(* Logix 5000 Routine export ReadAllSegStatus; software revision 20.04 *)

TYPE Segment_Status :
STRUCT
   Speed_pulse_status : BOOL; {access Read Only}
   Exists : BOOL; {access Read Only}
   Group_number : INT; {access Read Only}
END_STRUCT
END_TYPE

VAR_GLOBAL   (* controller tags *)
   Status_of_Segments : Segment_Status[50]; {access Read Only}
END_VAR

PROGRAM MainProgram

ROUTINE ReadAllSegStatus   (* ladder *)
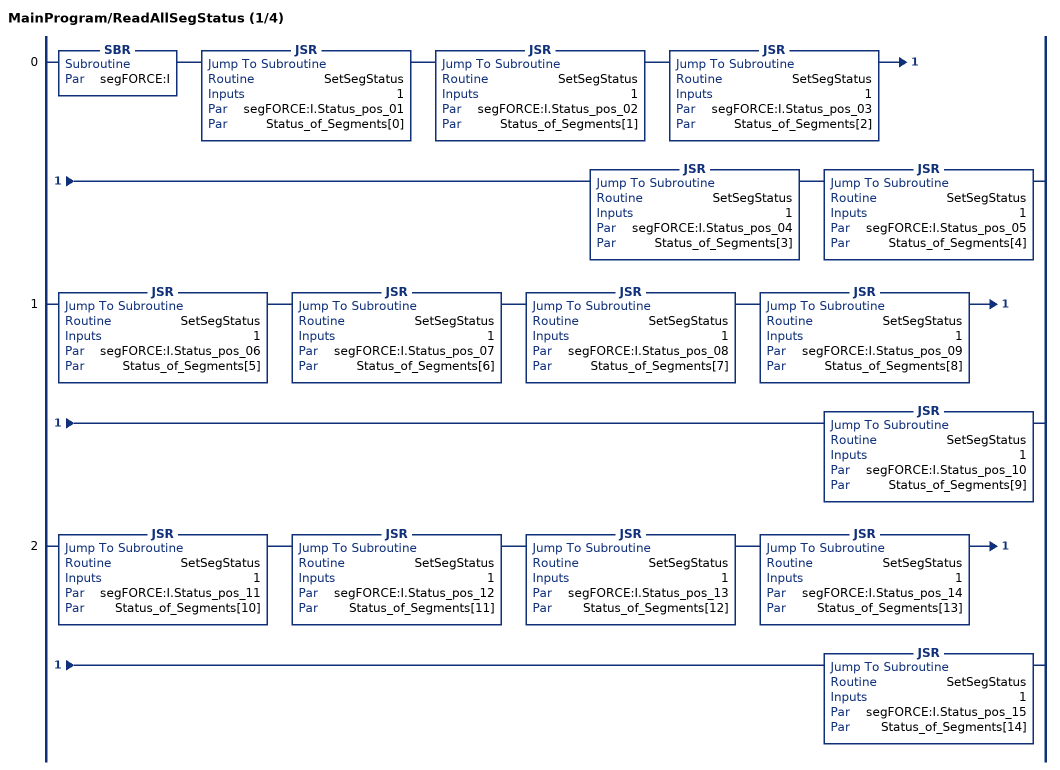
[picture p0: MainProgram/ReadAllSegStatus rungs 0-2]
   0: SBR(segFORCE:I)JSR(SetSegStatus,1,segFORCE:I.Status_pos_01,Status_of_Segments[0])JSR(SetSegStatus,1,segFORCE:I.Status_pos_02,Status_of_Segments[1])JSR(SetSegStatus,1,segFORCE:I.Status_pos_03,Status_of_Segments[2])JSR(SetSegStatus,1,segFORCE:I.Status_pos_04,Status_of_Segments[3])JSR(SetSegStatus,1,segFORCE:I.Status_pos_05,Status_of_Segments[4]);
   1: JSR(SetSegStatus,1,segFORCE:I.Status_pos_06,Status_of_Segments[5])JSR(SetSegStatus,1,segFORCE:I.Status_pos_07,Status_of_Segments[6])JSR(SetSegStatus,1,segFORCE:I.Status_pos_08,Status_of_Segments[7])JSR(SetSegStatus,1,segFORCE:I.Status_pos_09,Status_of_Segments[8])JSR(SetSegStatus,1,segFORCE:I.Status_pos_10,Status_of_Segments[9]);
   2: JSR(SetSegStatus,1,segFORCE:I.Status_pos_11,Status_of_Segments[10])JSR(SetSegStatus,1,segFORCE:I.Status_pos_12,Status_of_Segments[11])JSR(SetSegStatus,1,segFORCE:I.Status_pos_13,Status_of_Segments[12])JSR(SetSegStatus,1,segFORCE:I.Status_pos_14,Status_of_Segments[13])JSR(SetSegStatus,1,segFORCE:I.Status_pos_15,Status_of_Segments[14]);
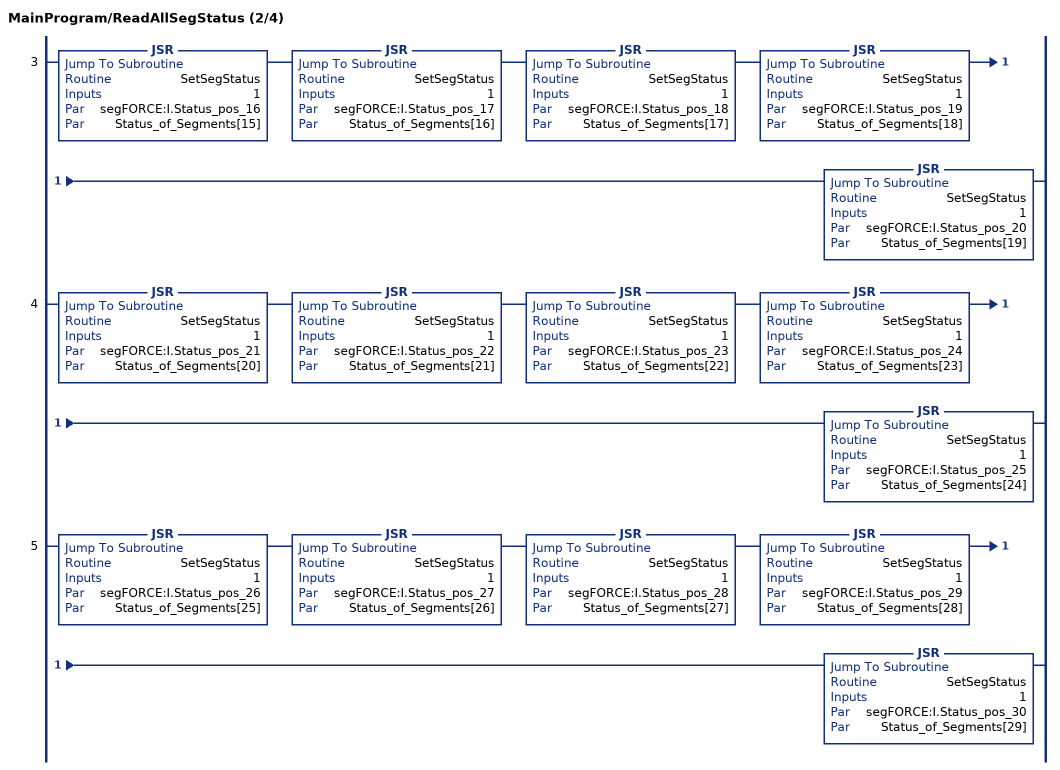
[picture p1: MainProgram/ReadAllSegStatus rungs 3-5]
   3: JSR(SetSegStatus,1,segFORCE:I.Status_pos_16,Status_of_Segments[15])JSR(SetSegStatus,1,segFORCE:I.Status_pos_17,Status_of_Segments[16])JSR(SetSegStatus,1,segFORCE:I.Status_pos_18,Status_of_Segments[17])JSR(SetSegStatus,1,segFORCE:I.Status_pos_19,Status_of_Segments[18])JSR(SetSegStatus,1,segFORCE:I.Status_pos_20,Status_of_Segments[19]);
   4: JSR(SetSegStatus,1,segFORCE:I.Status_pos_21,Status_of_Segments[20])JSR(SetSegStatus,1,segFORCE:I.Status_pos_22,Status_of_Segments[21])JSR(SetSegStatus,1,segFORCE:I.Status_pos_23,Status_of_Segments[22])JSR(SetSegStatus,1,segFORCE:I.Status_pos_24,Status_of_Segments[23])JSR(SetSegStatus,1,segFORCE:I.Status_pos_25,Status_of_Segments[24]);
   5: JSR(SetSegStatus,1,segFORCE:I.Status_pos_26,Status_of_Segments[25])JSR(SetSegStatus,1,segFORCE:I.Status_pos_27,Status_of_Segments[26])JSR(SetSegStatus,1,segFORCE:I.Status_pos_28,Status_of_Segments[27])JSR(SetSegStatus,1,segFORCE:I.Status_pos_29,Status_of_Segments[28])JSR(SetSegStatus,1,segFORCE:I.Status_pos_30,Status_of_Segments[29]);
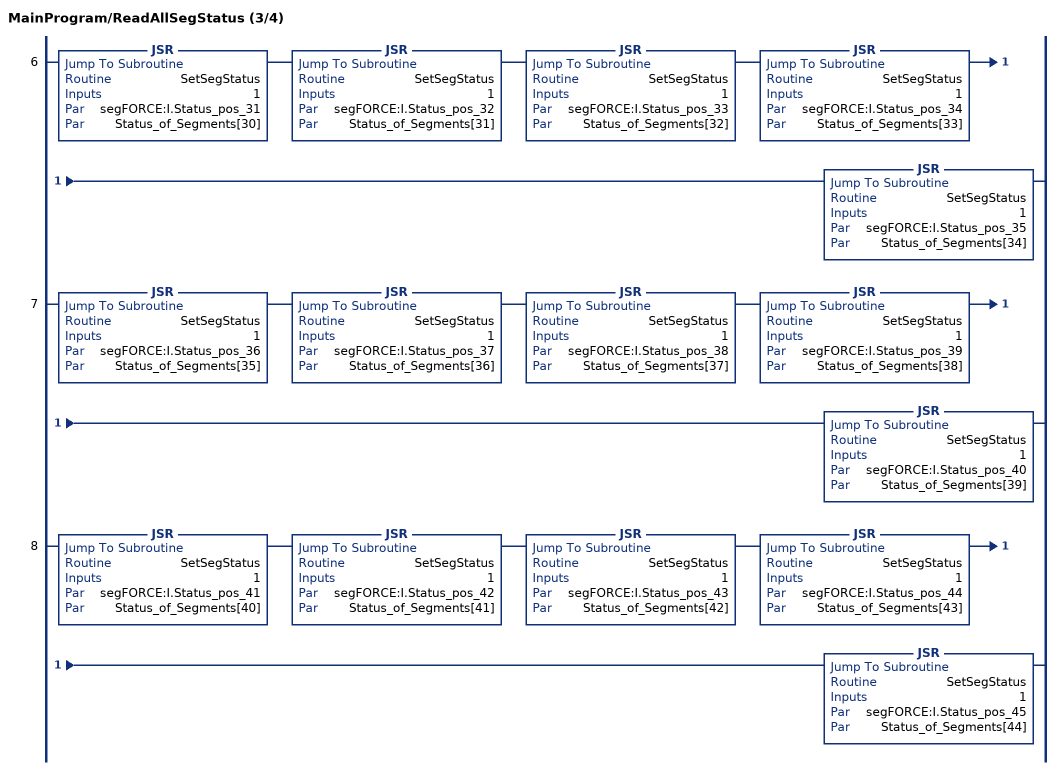
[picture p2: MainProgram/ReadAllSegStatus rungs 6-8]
   6: JSR(SetSegStatus,1,segFORCE:I.Status_pos_31,Status_of_Segments[30])JSR(SetSegStatus,1,segFORCE:I.Status_pos_32,Status_of_Segments[31])JSR(SetSegStatus,1,segFORCE:I.Status_pos_33,Status_of_Segments[32])JSR(SetSegStatus,1,segFORCE:I.Status_pos_34,Status_of_Segments[33])JSR(SetSegStatus,1,segFORCE:I.Status_pos_35,Status_of_Segments[34]);
   7: JSR(SetSegStatus,1,segFORCE:I.Status_pos_36,Status_of_Segments[35])JSR(SetSegStatus,1,segFORCE:I.Status_pos_37,Status_of_Segments[36])JSR(SetSegStatus,1,segFORCE:I.Status_pos_38,Status_of_Segments[37])JSR(SetSegStatus,1,segFORCE:I.Status_pos_39,Status_of_Segments[38])JSR(SetSegStatus,1,segFORCE:I.Status_pos_40,Status_of_Segments[39]);
   8: JSR(SetSegStatus,1,segFORCE:I.Status_pos_41,Status_of_Segments[40])JSR(SetSegStatus,1,segFORCE:I.Status_pos_42,Status_of_Segments[41])JSR(SetSegStatus,1,segFORCE:I.Status_pos_43,Status_of_Segments[42])JSR(SetSegStatus,1,segFORCE:I.Status_pos_44,Status_of_Segments[43])JSR(SetSegStatus,1,segFORCE:I.Status_pos_45,Status_of_Segments[44]);
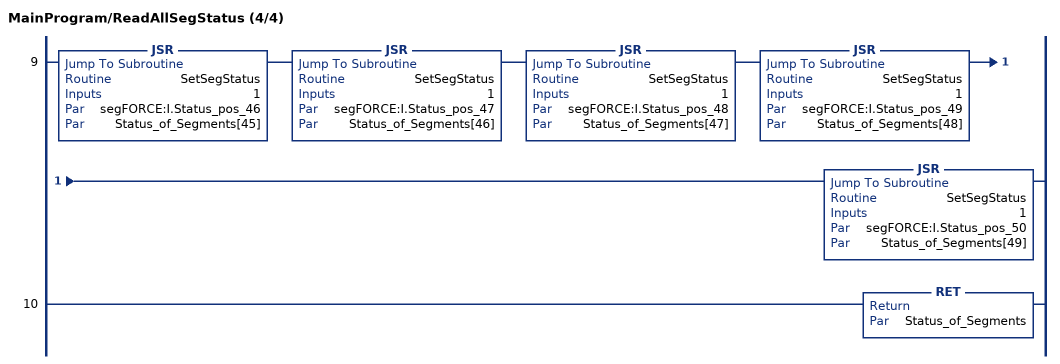
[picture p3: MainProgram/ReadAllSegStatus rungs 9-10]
   9: JSR(SetSegStatus,1,segFORCE:I.Status_pos_46,Status_of_Segments[45])JSR(SetSegStatus,1,segFORCE:I.Status_pos_47,Status_of_Segments[46])JSR(SetSegStatus,1,segFORCE:I.Status_pos_48,Status_of_Segments[47])JSR(SetSegStatus,1,segFORCE:I.Status_pos_49,Status_of_Segments[48])JSR(SetSegStatus,1,segFORCE:I.Status_pos_50,Status_of_Segments[49]);
   10: RET(Status_of_Segments);
END_ROUTINE
END_PROGRAM
